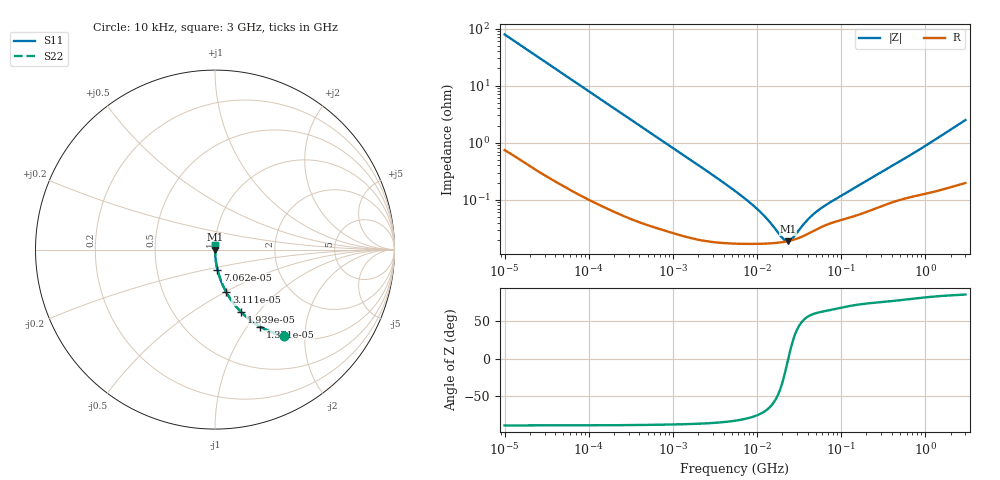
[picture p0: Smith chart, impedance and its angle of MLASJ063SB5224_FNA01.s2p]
! MLASJ063SB5224_FNA01  S-PARAMETER MODEL  ( Standard Model )
! Model Generated by TAIYO YUDEN Corporation (http://www.ty-top.com)
! Version 1.0
! TAIYO YUDEN Control No. 220601
! Copyright(c) 2006 TAIYO YUDEN CO.,LTD. All Rights Reserved.
! Product Description (link to TY-COMPAS)
! https://ds.yuden.co.jp/TYCOMPAS/or/detail?pn=MLASJ063SB5224KFNA01&u=M
! Products Name : Multilayer Ceramic Capacitors
! Characteristics :
!  Capacitance : 0.22 [uF] , Rated Voltage : 6.3 [V] , TCC : X5R
!  Case Size : 0.6 x 0.3 / 0.024 x 0.012 [mm/inch] , Thickness : 0.3 / 0.012 [mm/inch]
!  (Conditions: Temperature = 25 [degC] , DC Bias Voltage = 0 [V])
! External Node Assignments :
!  1  o---| |---o  2
! GND o---------o GND
! Frequency Range : 10kHz  -  3GHz  [ 401 STEP ]
# MHZ S RI R 50
! Freq[MHz].  S11 Real  S11 Imag  S21 Real  S21 Imag  S12 Real  S12 Imag  S22 Real  S22 Imag
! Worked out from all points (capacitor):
!   401 points, 10 kHz to 3 GHz, reference 50 ohm
!   read as one part in series: C = 202 nF near 10.65 kHz
!   lowest |Z| = 18.9 mohm at 23.36 MHz (marker M1)
!   series resonance near 23.58 MHz, so ESL is about 230 pH
!   S11 on the Smith chart (normalised r, x): 10 kHz: 1.01, -1.57; 13.71 kHz: 1.01, -1.15; 19.39 kHz: 1.01, -0.82; 31.11 kHz: 1.01, -0.51; 70.62 kHz: 1.00, -0.23; 3 GHz: 1.00, +0.05
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0.01  0.3837 -0.4816  0.6163 0.4816  0.6163 0.4816  0.3837 -0.4816
0.013707  0.251 -0.4288  0.749 0.4288  0.749 0.4288  0.251 -0.4288
0.019389  0.1451 -0.3473  0.8549 0.3473  0.8549 0.3473  0.1451 -0.3473
0.031113  0.0631 -0.2382  0.9369 0.2382  0.9369 0.2382  0.0631 -0.2382
0.046876  0.0296 -0.1643  0.9704 0.1643  0.9704 0.1643  0.0296 -0.1643
0.070624  0.0138 -0.1111  0.9862 0.1111  0.9862 0.1111  0.0138 -0.1111
0.082683  0.0103 -0.0954  0.9897 0.0954  0.9897 0.0954  0.0103 -0.0954
0.199902  0.00222 -0.04  0.9978 0.04  0.9978 0.04  0.00222 -0.04
0.683653  0.000451 -0.0118  0.9995 0.0118  0.9995 0.0118  0.000451 -0.0118
5.477226  0.000173 -0.00142  0.9998 0.00142  0.9998 0.00142  0.000173 -0.00142
10.29003  0.00017 -0.000647  0.9998 0.000647  0.9998 0.000647  0.00017 -0.000647
13.66633  0.000172 -0.0004  0.9998 0.0004  0.9998 0.0004  0.000172 -0.0004
19.95104  0.000181 -0.000117  0.9998 0.000117  0.9998 0.000117  0.000181 -0.000117
21.93027  0.000185 -5.04e-05  0.9998 5.04e-05  0.9998 5.04e-05  0.000185 -5.04e-05
23.35767  0.000189 -6.41e-06  0.9998 6.41e-06  0.9998 6.41e-06  0.000189 -6.41e-06
26.49725  0.000198 8.13e-05  0.9998 -8.13e-05  0.9998 -8.13e-05  0.000198 8.13e-05
36.31858  0.000235 0.000302  0.9998 -0.000302  0.9998 -0.000302  0.000235 0.000302
45.28751  0.000277 0.000458  0.9997 -0.000458  0.9997 -0.000458  0.000277 0.000458
70.41703  0.000375 0.000777  0.9996 -0.000777  0.9996 -0.000777  0.000375 0.000777
374.4521  0.00088 0.00358  0.9991 -0.00358  0.9991 -0.00358  0.00088 0.00358
823.6  0.00125 0.00725  0.9988 -0.00725  0.9988 -0.00725  0.00125 0.00725
3000  0.00258 0.0247  0.9974 -0.0247  0.9974 -0.0247  0.00258 0.0247
